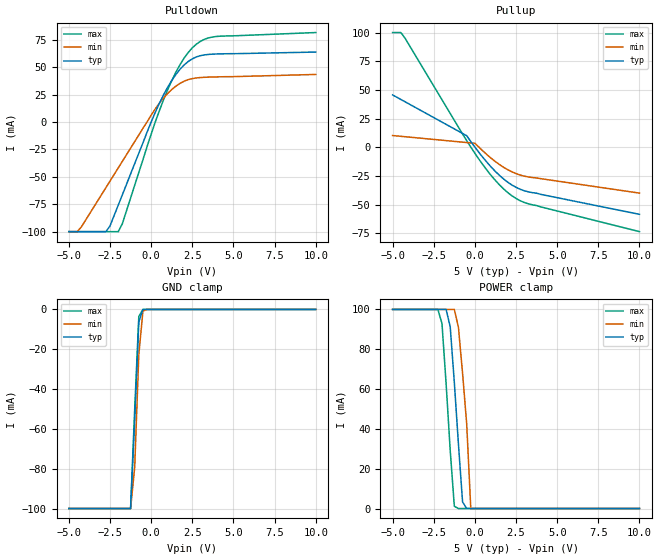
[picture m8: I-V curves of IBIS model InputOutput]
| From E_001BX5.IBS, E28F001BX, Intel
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|*******************Input Output Model********************************
[Model]   InputOutput
Model_type   I/O
|   Model for DQ[0:7]
Vinl = 0.8V
Vinh = 2.0V
|Variable   Typ   Min   Max
C_comp   10.00p   8.00p   12.00p
[Voltage Range]   5.0V   4.5V   5.5V
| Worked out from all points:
|   slope of the pulldown table from 0 to 0.75 V, typ, clamps not added: 30.5 ohm
|   slope of the pullup table from 0 to 0.75 V, typ, clamps not added: 55.5 ohm
|   GND clamp passes 1 mA (typ) near -0.54 V on its own axis
|   POWER clamp passes 1 mA (typ) near -0.58 V on its own axis
[Pulldown]
| [Pullup] and [Pulldown] IV curves include only the current through
| the channels of output driver transistors when outputs are enabled
| with OE# = VIL.  Although the output driver transistors have np and
| pn diodes inherently created by CMOS IC fabrication between the
| drain and bulk of n-channel and p-channel CMOS transistors,
| the current through these junction diodes is not included in
| [Pullup] or [Pulldown].  Instead that drain/bulk diode current is
| included in the [POWER_clamp] or [GND_clamp] sections, which are
| not dependent on the state of OE# or output data value.
|Voltage   I(typ)   I(min)   I(max)
-5V       -100mA     -100mA     -100mA
-4.5V     -100mA     -100mA     -100mA
-4.25V    -100mA     -95.9mA    -100mA
-2.75V    -100mA     -59.9mA    -100mA
-2.5V     -94.82mA   -53.9mA    -100mA
-2V       -75.87mA   -41.9mA    -100mA
-1.75V    -66.4mA    -35.9mA    -92.73mA
750mV     24.59mA    21.78mA    20.07mA
1.75V     47.93mA    35.13mA    52.14mA
2.75V     59.28mA    40.12mA    70.93mA
4V        61.97mA    41.07mA    77.96mA
10V       63.7mA     43.3mA     81.5mA
[GND_clamp]
| [POWER_clamp] and [GND_clamp] IV curves describe ESD protection
| circuits PLUS some np and pn diodes which exist between the
| drain and bulk of n-channel and p-channel CMOS transistors.
| These drain/bulk diodes are inherent in CMOS IC fabrication,
| and are visible on the node of the I/O pin at all times.
| Even the drain/bulk diodes of output driver [Pullup] and [Powerdown]
| transistors are included in [POWER_clamp] or [GND_clamp], because
| these diodes contribute to I/O pin current even when the
| chip outputs are tristated by OE# = VIH.
| For example, when V forced on the I/O pin is large, we are
| forward biasing the pn diode at the drain/bulk interface in the
| p-channel pullup transistor.  Similarly, when V forced on the
| I/O pin is sufficiently negative with respect to the substrate
| ground, we are forward biasing the np diode at the drain/bulk
| interface in the n-channel pulldown transistor.  The effects
| of these diodes are included in [POWER_clamp] or [GND_clamp].
|Voltage   I(typ)   I(min)   I(max)
-5V       -99.85mA   -99.84mA   -99.85mA
-1.25V    -99.85mA   -99.84mA   -99.85mA
-1V       -55.55mA   -79.12mA   -50.05mA
-750mV    -6.293mA   -22.64mA   -3.481mA
-500mV    -40.69uA   -915.2uA   -16.56uA
-250mV    0A         0A         0A
10V       0A         0A         0A
[Pullup]
| (Voltages for [Pullup] and [POWER_clamp] are specified with
| negative respect to Vcc.  Reference the IBIS documentation
| for more information regarding Vtable = Vcc - Voutput.
| This method keeps -Vds constant for the values in all three
| columns across a line of the table.
| [Pullup] and [Pulldown] IV curves include only the current through
| the channels of output driver transistors when outputs are enabled
| with OE# = VIL.  Although the output driver transistors have np and
| pn diodes inherently created by CMOS IC fabrication between the
| drain and bulk of n-channel and p-channel CMOS transistors,
| the current through these junction diodes is not included in
| [Pullup] or [Pulldown].  Instead that drain/bulk diode current is
| included in the [POWER_clamp] or [GND_clamp] sections, which are
| not dependent on the state of OE# or output data value.
|Voltage   I(typ)   I(min)   I(max)
-5V       45.6mA     10.2mA     100mA
-4.5V     41.65mA    9.52mA     100mA
-4.25V    39.68mA    9.18mA     95.18mA
-500mV    10.05mA    4.08mA     5.747mA
0V        77.16uA    3.439mA    -5.319mA
1V        -17.45mA   -9.768mA   -24.85mA
1.5V      -24.62mA   -15.18mA   -32.91mA
2V        -30.52mA   -19.62mA   -39.57mA
2.5V      -34.98mA   -22.99mA   -44.67mA
3.25V     -38.91mA   -25.93mA   -49.35mA
10V       -58.5mA    -40mA      -73.6mA
[POWER_clamp]
| (Voltages for [Pullup] and [POWER_clamp] are specified with
| negative respect to Vcc.  Reference the IBIS documentation
| for more information regarding Vtable = Vcc - Voutput.
| This method keeps -Vds constant for the values in all three
| columns across a line of the table.
| [POWER_clamp] and [GND_clamp] IV curves describe ESD protection
| circuits PLUS some np and pn diodes which exist between the
| drain and bulk of n-channel and p-channel CMOS transistors.
| These drain/bulk diodes are inherent in CMOS IC fabrication,
| and are visible on the node of the I/O pin at all times.
| Even the drain/bulk diodes of output driver [Pullup] and [Powerdown]
| transistors are included in [POWER_clamp] or [GND_clamp], because
| these diodes contribute to I/O pin current even when the
| chip outputs are tristated by OE# = VIH.
| For example, when V forced on the I/O pin is large, we are
| forward biasing the pn diode at the drain/bulk interface in the
| p-channel pullup transistor.  Similarly, when V forced on the
| I/O pin is sufficiently negative with respect to the substrate
| ground, we are forward biasing the np diode at the drain/bulk
| interface in the n-channel pulldown transistor.  The effects
| of these diodes are included in [POWER_clamp] or [GND_clamp].
|Voltage I(typ)   I(min)   I(max)
-5V       100mA      100mA      100mA
-2.25V    100mA      100mA      100mA
-2V       100mA      100mA      92.85mA
-1.75V    100mA      100mA      62.76mA
-1.5V     91.27mA    100mA      29.19mA
-1.25V    63.32mA    100mA      1.12mA
-1V       32.35mA    90.99mA    49.41nA
-750mV    3.299mA    67.97mA    0A
-500mV    552.9nA    42.64mA    0A
-250mV    0A         0A         0A
10V       0A         0A         0A
[Ramp]
| The DQ Ramp information is not provided at this time for the
| device but will be available in the future.  The table below
| is for the compatibility with some IBIS parsers.
| Variable   typ   min   max
 dV/dt_r   0V/0ns   0V/0ns   0V/0ns
 dV/dt_f   0V/0ns   0V/0ns   0V/0ns
